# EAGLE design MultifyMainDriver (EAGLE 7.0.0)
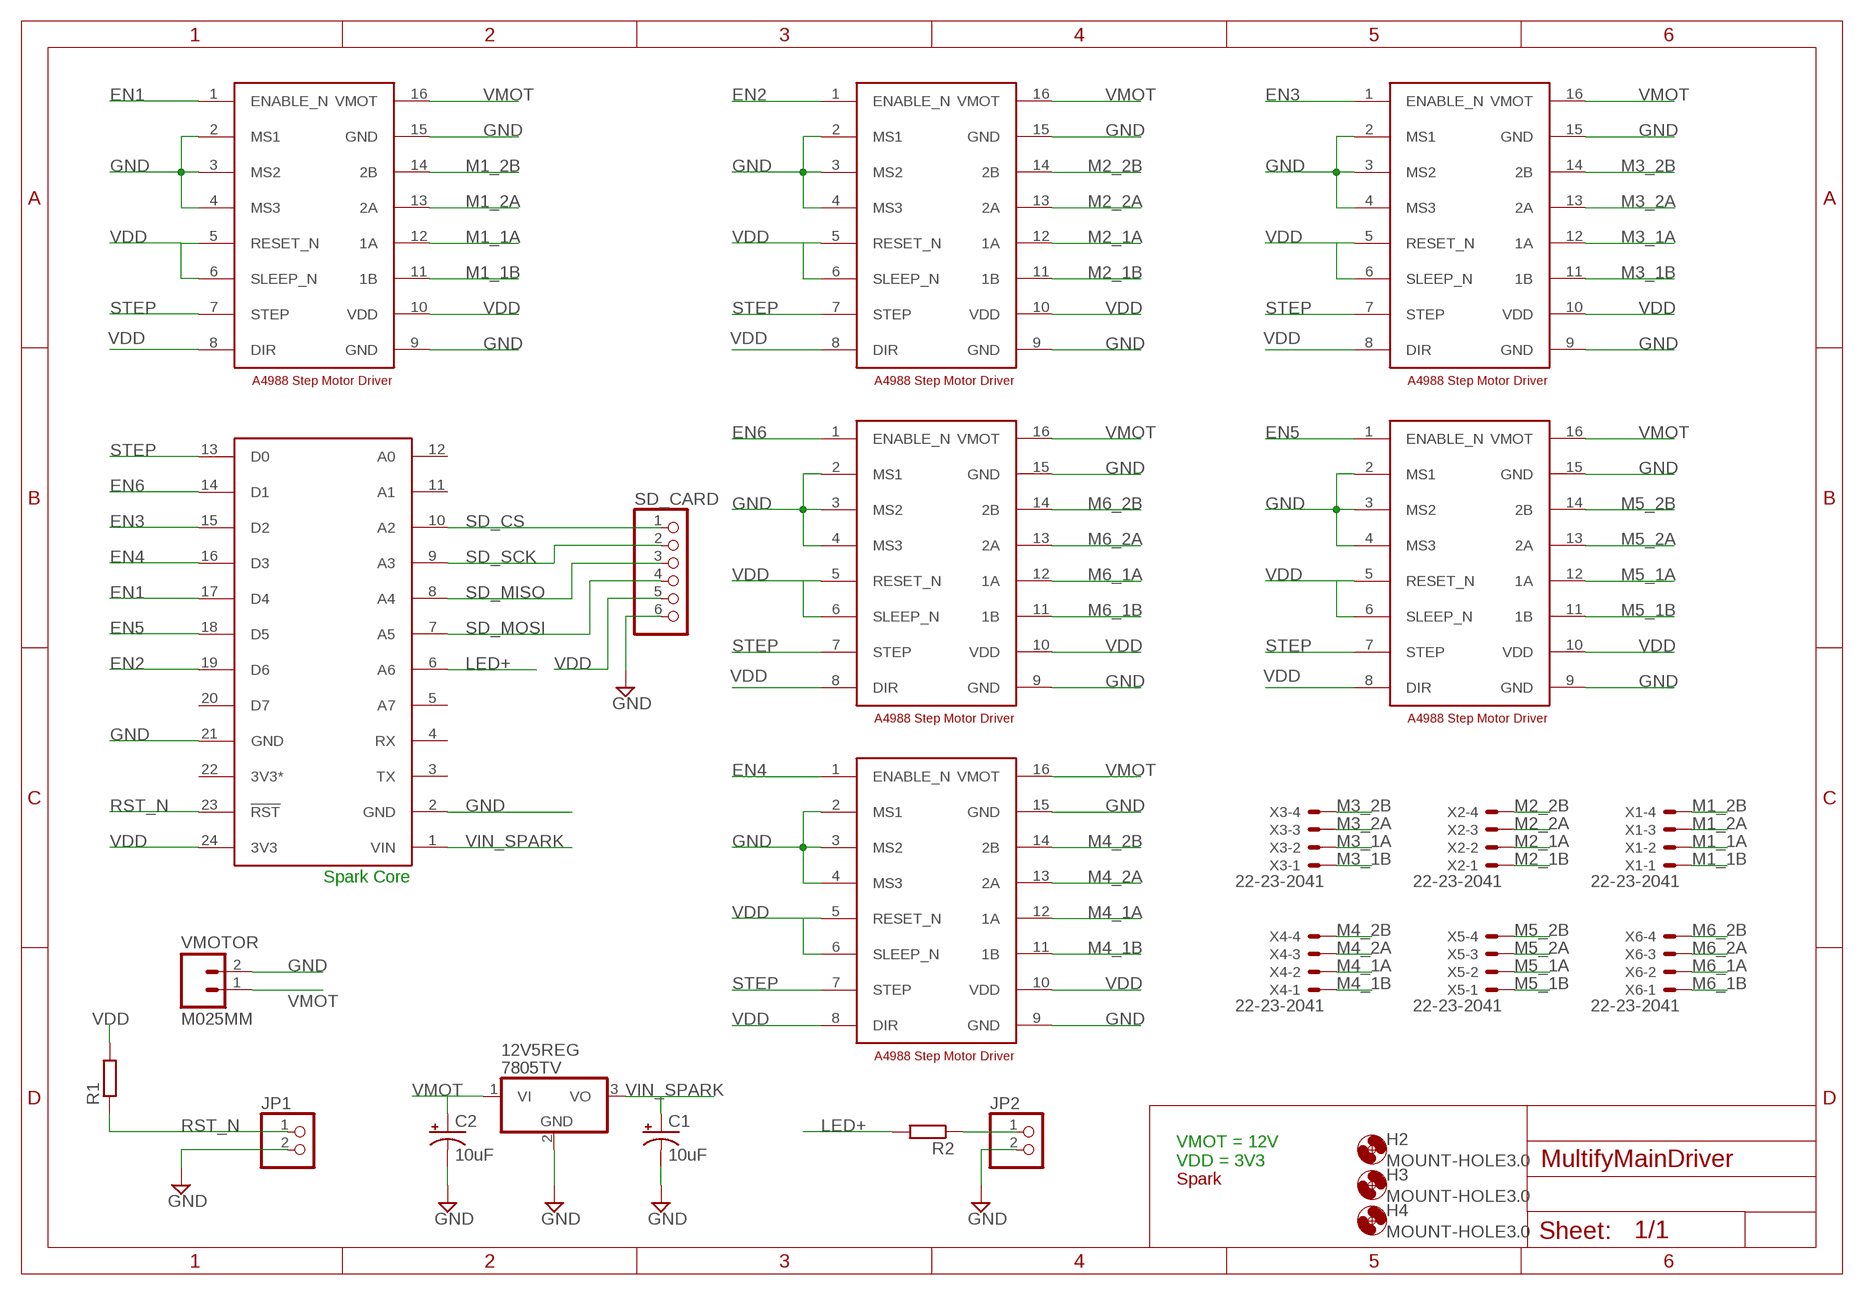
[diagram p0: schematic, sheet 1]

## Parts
12V5REG  7805TV  [TO220V]
C1  10uF  CPOL-USE3.5-8  [E3,5-8]
C2  10uF  CPOL-USE3.5-8  [E3,5-8]
DRIVER1  A4988_DEV  [A4988_PAC]
DRIVER2  A4988_DEV  [A4988_PAC]
DRIVER3  A4988_DEV  [A4988_PAC]
DRIVER4  A4988_DEV  [A4988_PAC]
DRIVER5  A4988_DEV  [A4988_PAC]
DRIVER6  A4988_DEV  [A4988_PAC]
H2  MOUNT-HOLE3.0  [3,0]
H3  MOUNT-HOLE3.0  [3,0]
H4  MOUNT-HOLE3.0  [3,0]
JP1  PINHD-1X2  [1X02]
JP2  PINHD-1X2  [1X02]
R1  R-EU_0207/7  [0207/7]
R2  R-EU_0207/7  [0207/7]
SD_CARD  PINHD-1X6  [1X06]
SPARK  SPARK_CORECORE  [SPARK_CORE]
U$2  SPARK_LOGO_WITH_PLANE  [SPARK_LOGO_PLUS_PLANE]
VMOTOR  M025MM  [SCREWTERMINAL-5MM-2]
X1  22-23-2041  [22-23-2041]
X2  22-23-2041  [22-23-2041]
X3  22-23-2041  [22-23-2041]
X4  22-23-2041  [22-23-2041]
X5  22-23-2041  [22-23-2041]
X6  22-23-2041  [22-23-2041]

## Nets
EN1: DRIVER1.1(ENABLE_N) SPARK.17(D4)
EN2: DRIVER2.1(ENABLE_N) SPARK.19(D6)
EN3: DRIVER3.1(ENABLE_N) SPARK.15(D2)
EN4: DRIVER4.1(ENABLE_N) SPARK.16(D3)
EN5: DRIVER6.1(ENABLE_N) SPARK.18(D5)
EN6: DRIVER5.1(ENABLE_N) SPARK.14(D1)
GND: 12V5REG.2(GND) C1.- C2.- DRIVER1.2(MS1) DRIVER1.3(MS2) DRIVER1.4(MS3) DRIVER1.9(GND) DRIVER1.15(GND) DRIVER2.2(MS1) DRIVER2.3(MS2) DRIVER2.4(MS3) DRIVER2.9(GND) DRIVER2.15(GND) DRIVER3.2(MS1) DRIVER3.3(MS2) DRIVER3.4(MS3) DRIVER3.9(GND) DRIVER3.15(GND) DRIVER4.2(MS1) DRIVER4.3(MS2) DRIVER4.4(MS3) DRIVER4.9(GND) DRIVER4.15(GND) DRIVER5.2(MS1) DRIVER5.3(MS2) DRIVER5.4(MS3) DRIVER5.9(GND) DRIVER5.15(GND) DRIVER6.2(MS1) DRIVER6.3(MS2) DRIVER6.4(MS3) DRIVER6.9(GND) DRIVER6.15(GND) JP1.2 JP2.2 SD_CARD.6 SPARK.2(GND) SPARK.21(GND) VMOTOR.2
LED+: R2.2 SPARK.6(A6)
M1_1A: DRIVER1.12(1A) X1.2
M1_1B: DRIVER1.11(1B) X1.1
M1_2A: DRIVER1.13(2A) X1.3
M1_2B: DRIVER1.14(2B) X1.4
M2_1A: DRIVER2.12(1A) X2.2
M2_1B: DRIVER2.11(1B) X2.1
M2_2A: DRIVER2.13(2A) X2.3
M2_2B: DRIVER2.14(2B) X2.4
M3_1A: DRIVER3.12(1A) X3.2
M3_1B: DRIVER3.11(1B) X3.1
M3_2A: DRIVER3.13(2A) X3.3
M3_2B: DRIVER3.14(2B) X3.4
M4_1A: DRIVER4.12(1A) X4.2
M4_1B: DRIVER4.11(1B) X4.1
M4_2A: DRIVER4.13(2A) X4.3
M4_2B: DRIVER4.14(2B) X4.4
M5_1A: DRIVER6.12(1A) X5.2
M5_1B: DRIVER6.11(1B) X5.1
M5_2A: DRIVER6.13(2A) X5.3
M5_2B: DRIVER6.14(2B) X5.4
M6_1A: DRIVER5.12(1A) X6.2
M6_1B: DRIVER5.11(1B) X6.1
M6_2A: DRIVER5.13(2A) X6.3
M6_2B: DRIVER5.14(2B) X6.4
N$1: JP2.1 R2.1
RST_N: JP1.1 R1.1 SPARK.23(!RST)
SD_CS: SD_CARD.1 SPARK.10(A2)
SD_MISO: SD_CARD.3 SPARK.8(A4)
SD_MOSI: SD_CARD.4 SPARK.7(A5)
SD_SCK: SD_CARD.2 SPARK.9(A3)
STEP: DRIVER1.7(STEP) DRIVER2.7(STEP) DRIVER3.7(STEP) DRIVER4.7(STEP) DRIVER5.7(STEP) DRIVER6.7(STEP) SPARK.13(D0)
VDD: DRIVER1.5(RESET_N) DRIVER1.6(SLEEP_N) DRIVER1.8(DIR) DRIVER1.10(VDD) DRIVER2.5(RESET_N) DRIVER2.6(SLEEP_N) DRIVER2.8(DIR) DRIVER2.10(VDD) DRIVER3.5(RESET_N) DRIVER3.6(SLEEP_N) DRIVER3.8(DIR) DRIVER3.10(VDD) DRIVER4.5(RESET_N) DRIVER4.6(SLEEP_N) DRIVER4.8(DIR) DRIVER4.10(VDD) DRIVER5.5(RESET_N) DRIVER5.6(SLEEP_N) DRIVER5.8(DIR) DRIVER5.10(VDD) DRIVER6.5(RESET_N) DRIVER6.6(SLEEP_N) DRIVER6.8(DIR) DRIVER6.10(VDD) R1.2 SD_CARD.5 SPARK.24(3V3)
VIN_SPARK: 12V5REG.3(VO) C1.+ SPARK.1(VIN)
VMOT: 12V5REG.1(VI) C2.+ DRIVER1.16(VMOT) DRIVER2.16(VMOT) DRIVER3.16(VMOT) DRIVER4.16(VMOT) DRIVER5.16(VMOT) DRIVER6.16(VMOT) VMOTOR.1
Unconnected: SPARK.3(TX) SPARK.4(RX) SPARK.5(A7) SPARK.11(A1) SPARK.12(A0) SPARK.20(D7)

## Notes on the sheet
- Spark Core
- VMOT = 12V
  VDD = 3V3

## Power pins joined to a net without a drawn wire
3V3*: SPARK.22(3V3*)

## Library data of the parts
12V5REG = linear:78*: Positive VOLTAGE REGULATOR Source: http://cache.national.com/ds/LM/LM78L05.pdf http://www.fairchildsemi.com/ds/LM/LM7805.pdf
C1 C2 = rcl:CPOL-US: POLARIZED CAPACITOR, American symbol
DRIVER1-DRIVER6 = A4988:A4988_DEV
H2-H4 = holes:MOUNT-HOLE: MOUNTING HOLE with drill center marker
JP1 JP2 = pinhead:PINHD-1X2: PIN HEADER
R1 R2 = rcl:R-EU_: RESISTOR, European symbol
SD_CARD = pinhead:PINHD-1X6: PIN HEADER
SPARK = Spark:SPARK_CORE
U$2 = Spark:SPARK_LOGO_WITH_PLANE
VMOTOR = SparkFun-Connectors:M02: Standard 2-pin 0.1" header. Use with; STOREFRONT_ID: PRT-08432
X1-X6 = con-molex:22-23-2041: .100" (2.54mm) Center Header - 4 Pin; MF: MOLEX; MPN: 22-23-2041; OC_FARNELL: 1462920; OC_NEWARK: 38C0355

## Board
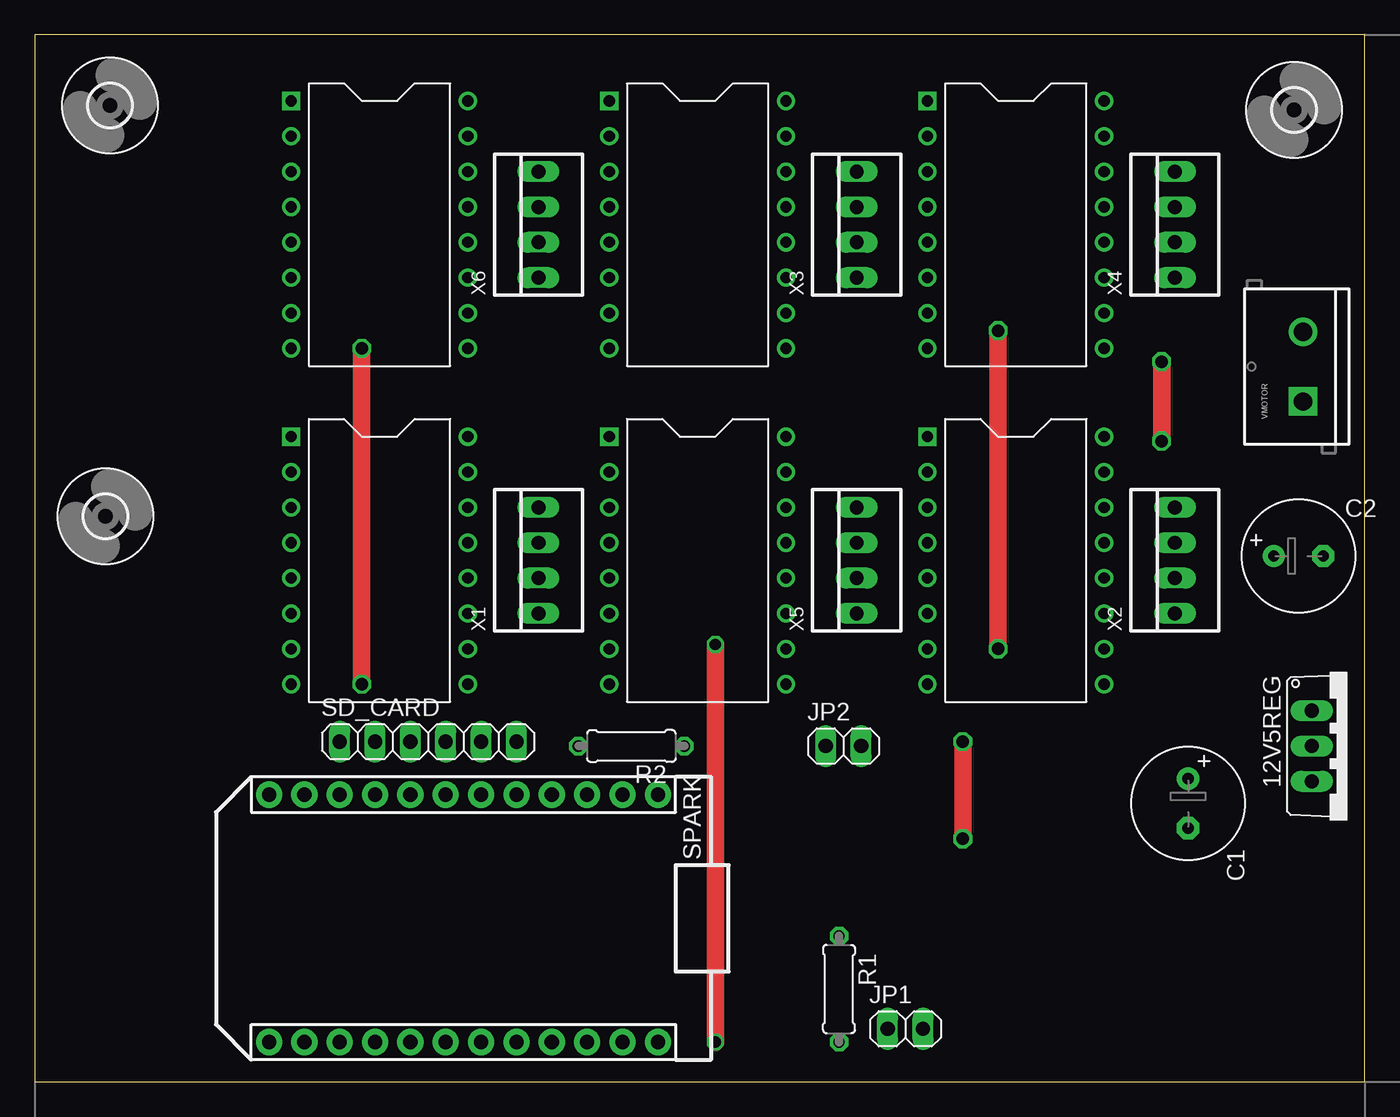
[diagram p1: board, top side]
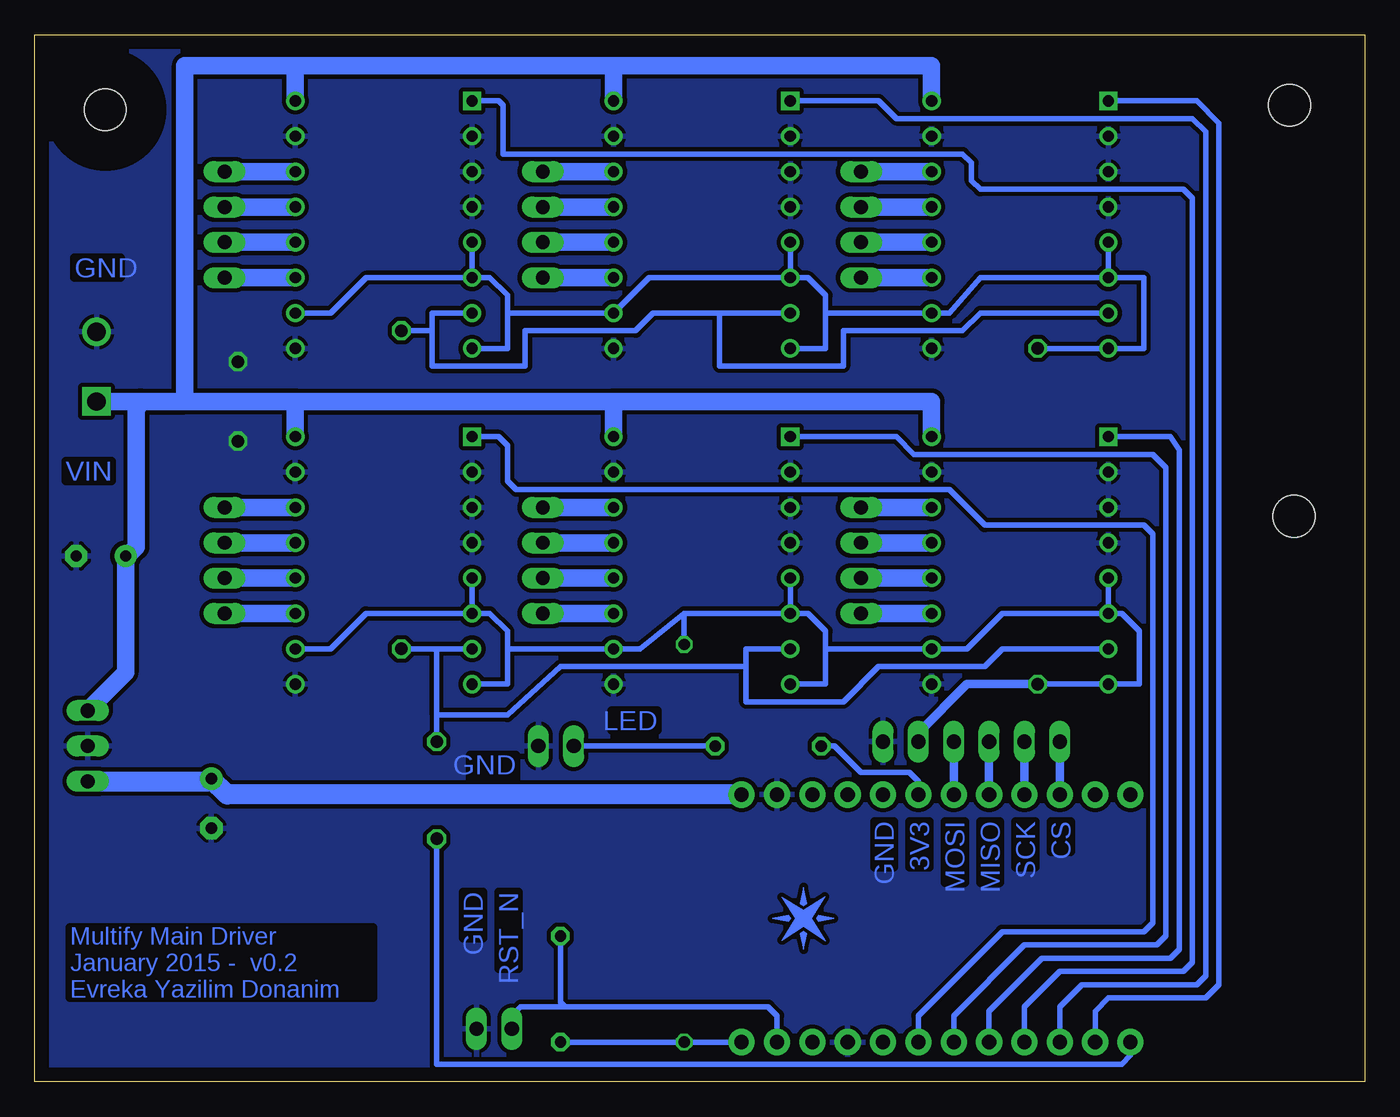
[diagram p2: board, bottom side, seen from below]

Size 95.56 x 75.24 mm. Coordinates in mm from the lower left corner, seen from the top.
Outline: 0,0 95.56,0 95.56,75.24 0,75.24 0,0
Copper layers (1*16): Top 0.035mm / dielectric 1.5mm / Bottom 0.035mm
Design rules "default": minimum track width 10mil, minimum drill 24mil, track to track 8mil, track to pad 8mil, pad to pad 8mil, via to via 8mil, smd to smd 8mil, copper to edge 40mil, drill to drill 8mil, minimum pad ring 10mil, minimum via ring 8mil, stop-mask expansion 4mil, vias tented up to drill 0mil, thermal gap 10mil

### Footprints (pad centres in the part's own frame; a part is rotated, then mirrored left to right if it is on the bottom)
TO220V = drill 1.016 long: 1 -2.54,-2.54; 2 0,-2.54; 3 2.54,-2.54
E3,5-8 = drill 0.813 pad 1.6: + -1.778,0 | drill 0.813 pad 1.6 octagon: - 1.778,0
A4988_PAC = drill 0.8 square: 1 -6.35,8.89 | drill 0.8: 2 -6.35,6.35; 3 -6.35,3.81; 4 -6.35,1.27; 5 -6.35,-1.27; 6 -6.35,-3.81; 7 -6.35,-6.35; 8 -6.35,-8.89; 9 6.35,-8.89; 10 6.35,-6.35; 11 6.35,-3.81; 12 6.35,-1.27; 13 6.35,1.27; 14 6.35,3.81; 15 6.35,6.35; 16 6.35,8.89
3,0 = hole 3: 0,0
1X02 = drill 1.016 long: 1 -1.27,0; 2 1.27,0
0207/7 = drill 0.813 octagon: 1 -3.81,0; 2 3.81,0
1X06 = drill 1.016 long: 1 -6.35,0; 2 -3.81,0; 3 -1.27,0; 4 1.27,0; 5 3.81,0; 6 6.35,0
SPARK_CORE = drill 1.016 pad 1.88: 1 -8.89,13.97; 2 -8.89,11.43; 3 -8.89,8.89; 4 -8.89,6.35; 5 -8.89,3.81; 6 -8.89,1.27; 7 -8.89,-1.27; 8 -8.89,-3.81; 9 -8.89,-6.35; 10 -8.89,-8.89; 11 -8.89,-11.43; 12 -8.89,-13.97; 13 8.89,-13.97; 14 8.89,-11.43; 15 8.89,-8.89; 16 8.89,-6.35; 17 8.89,-3.81; 18 8.89,-1.27; 19 8.89,1.27; 20 8.89,3.81; 21 8.89,6.35; 22 8.89,8.89; 23 8.89,11.43; 24 8.89,13.97
SCREWTERMINAL-5MM-2 = drill 1.3 pad 2.032 square: 1 0,0 | drill 1.3 pad 2.032: 2 5,0
22-23-2041 = drill 1 long: 1 -3.81,0; 2 -1.27,0; 3 1.27,0; 4 3.81,0

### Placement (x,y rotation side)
12V5REG  94.3,24.13 270 top
C1  82.87,20 270 top
C2  90.81,37.78 0 top
DRIVER1  24.77,37.47 0 top
DRIVER2  70.48,37.47 0 top
DRIVER3  47.62,61.59 0 top
DRIVER4  70.48,61.59 0 top
DRIVER5  24.77,61.59 0 top
DRIVER6  47.62,37.47 0 top
H2  90.49,69.85 0 top
H3  5.08,40.64 0 top
H4  5.4,70.17 0 top
JP1  62.55,3.81 0 top
JP2  58.1,24.13 0 top
R1  57.78,6.67 270 top
R2  42.86,24.13 180 top
SD_CARD  28.26,24.45 0 top
SPARK  30.8,11.75 270 top
U$2  40.32,11.75 0 bottom
VMOTOR  91.12,48.9 90 top
X1  36.2,37.47 90 top
X2  81.92,37.47 90 top
X3  59.05,61.59 90 top
X4  81.92,61.59 90 top
X5  59.05,37.47 90 top
X6  36.2,61.59 90 top

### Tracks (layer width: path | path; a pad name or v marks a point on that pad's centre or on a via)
EN1
  Bottom 0.406: DRIVER1.1 13.97,46.35 13.34,45.4 13.34,9.53 13.97,8.89 23.18,8.89 26.99,5.08 SPARK.17
EN2
  Bottom 0.406: SPARK.19 32.07,4.76 26.04,10.79 15.88,10.79 15.24,11.43 15.24,39.37 15.88,40.01 27.3,40.01 29.84,42.55 60.96,42.55 61.59,43.18 61.59,45.72 62.23,46.35 DRIVER2.1
EN3
  Bottom 0.406: DRIVER3.1 34.92,70.48 33.66,69.22 12.38,69.22 11.43,68.26 11.43,7.62 12.06,6.99 20.32,6.99 21.91,5.4 SPARK.15
EN4
  Bottom 0.406: DRIVER4.1 62.23,70.48 61.91,70.17 61.91,66.67 28.89,66.67 28.26,66.04 28.26,64.77 27.62,64.14 13.02,64.14 12.38,63.5 12.38,8.57 13.02,7.94 21.91,7.94 24.45,5.4 SPARK.16
EN5
  Bottom 0.406: DRIVER6.1 33.66,46.35 32.38,45.09 15.24,45.09 14.29,44.13 14.29,10.48 14.92,9.84 24.45,9.84 29.53,4.76 SPARK.18
EN6
  Bottom 0.406: 14.61,70.48 DRIVER5.1 12.06,70.48 10.48,68.9 10.48,6.99 11.43,6.03 18.41,6.03 19.37,5.08 SPARK.14
GND  (via drill 0.9)
  Top 1.27: v80.96,51.75 v80.96,46.04
  pour Bottom (isolate 0.305): 0.32,75.25 95.57,75.25 95.57,0 0.32,0
LED+
  Bottom 0.406: SPARK.6 32.07,21.59 32.7,22.23 36.2,22.23 38.1,24.13 R2.2
M1_1A
  Bottom 1.27: X1.2 DRIVER1.12
M1_1B
  Bottom 1.27: X1.1 DRIVER1.11
M1_2A
  Bottom 1.27: X1.3 DRIVER1.13
M1_2B
  Bottom 1.27: DRIVER1.14 X1.4
M2_1A
  Bottom 1.27: X2.2 DRIVER2.12
M2_1B
  Bottom 1.27: X2.1 DRIVER2.11
M2_2A
  Bottom 1.27: X2.3 DRIVER2.13
M2_2B
  Bottom 1.27: X2.4 DRIVER2.14
M3_1A
  Bottom 1.27: X3.2 DRIVER3.12
M3_1B
  Bottom 1.27: X3.1 DRIVER3.11
M3_2A
  Bottom 1.27: X3.3 DRIVER3.13
M3_2B
  Bottom 1.27: X3.4 DRIVER3.14
M4_1A
  Bottom 1.27: X4.2 DRIVER4.12
M4_1B
  Bottom 1.27: X4.1 DRIVER4.11
M4_2A
  Bottom 1.27: X4.3 DRIVER4.13
M4_2B
  Bottom 1.27: X4.4 DRIVER4.14
M5_1A
  Bottom 1.27: X5.2 DRIVER6.12
M5_1B
  Bottom 1.27: X5.1 DRIVER6.11
M5_2A
  Bottom 1.27: X5.3 DRIVER6.13
M5_2B
  Bottom 1.27: X5.4 DRIVER6.14
M6_1A
  Bottom 1.27: DRIVER5.12 X6.2
M6_1B
  Bottom 1.27: DRIVER5.11 X6.1
M6_2A
  Bottom 1.27: DRIVER5.13 X6.3
M6_2B
  Bottom 1.27: DRIVER5.14 X6.4
N$1
  Bottom 0.406: R2.1 JP2.1
RST_N
  Bottom 0.406: SPARK.23 42.23,4.76 42.86,5.4 57.47,5.4 | 57.47,5.4 60.64,5.4 61.28,4.76 JP1.1 | R1.1 57.78,5.71 57.47,5.4
SD_CS
  Bottom 0.61: SD_CARD.1 SPARK.10
SD_MISO
  Bottom 0.61: SD_CARD.3 SPARK.8
SD_MOSI
  Bottom 0.61: SD_CARD.4 SPARK.7
SD_SCK
  Bottom 0.61: SD_CARD.2 SPARK.9
STEP  (via drill 0.9)
  Top 1.27: v69.22,31.11 v69.22,53.98 | v66.67,24.45 v66.67,17.46
  Bottom 0.406: DRIVER6.7 44.45,31.11 44.45,29.84 | DRIVER5.7 27.62,55.24 28.89,53.98 37.47,53.98 37.47,51.44 46.35,51.44 46.35,55.24 | DRIVER3.7 46.35,55.24 | 46.35,55.24 51.12,55.24 52.39,53.98 60.33,53.98 60.33,51.44 66.99,51.44 66.99,53.98 | DRIVER4.7 66.99,55.24 66.99,53.98 | DRIVER1.7 26.04,31.11 27.3,29.84 34.92,29.84 37.47,27.3 44.45,27.3 44.45,29.84 | 44.45,29.84 57.78,29.84 61.59,26.35 66.67,26.35 | 66.67,26.35 66.67,31.11 | DRIVER2.7 66.67,31.11 | 66.67,31.11 v69.22,31.11 | v69.22,53.98 66.99,53.98 | SPARK.13 16.83,1.91 17.46,1.27 66.67,1.27 v66.67,17.46 | 66.67,26.35 v66.67,24.45
VDD  (via drill 0.8, 0.9)
  Top 1.27: v23.5,28.57 v23.5,52.7 | v48.9,2.86 v48.9,31.43
  Bottom 0.406: DRIVER5.5 DRIVER5.6 | DRIVER3.5 DRIVER3.6 | DRIVER4.5 DRIVER4.6 | DRIVER1.5 DRIVER1.6 | DRIVER6.5 DRIVER6.6 | DRIVER2.6 DRIVER2.5 | DRIVER2.10 74.3,31.11 71.75,33.66 DRIVER2.6 | DRIVER5.6 27.62,57.78 29.84,55.24 DRIVER5.10 38.73,55.24 | DRIVER3.6 51.44,57.78 DRIVER3.10 61.59,55.24 | DRIVER4.6 71.75,57.78 74.3,55.24 DRIVER4.10 | DRIVER6.6 48.9,33.66 | 48.9,33.66 52.07,31.11 DRIVER6.10 61.59,31.11 | DRIVER1.6 26.04,33.66 28.57,31.11 DRIVER1.10 38.73,31.11 | DRIVER5.6 15.88,57.78 15.88,52.7 DRIVER5.8 v23.5,52.7 | DRIVER3.8 38.73,52.7 38.73,55.24 | 38.73,55.24 38.73,56.52 40.01,57.78 DRIVER3.6 | DRIVER4.8 61.59,52.7 61.59,55.24 | 61.59,55.24 61.59,56.52 62.87,57.78 DRIVER4.6 | DRIVER1.6 17.46,33.66 16.19,32.38 16.19,28.57 DRIVER1.8 v23.5,28.57 | DRIVER6.8 38.73,28.57 38.73,31.11 | 38.73,31.11 38.73,32.38 40.01,33.66 DRIVER6.6 | DRIVER2.8 61.59,28.57 61.59,31.11 | 61.59,31.11 61.59,32.38 62.87,33.66 DRIVER2.6 | v48.9,31.43 48.9,33.66 | SPARK.24 v48.9,2.86 R1.2
  Bottom 0.61: SD_CARD.5 32.07,25.08 28.57,28.57 v23.5,28.57
VIN_SPARK
  Bottom 1.422: SPARK.1 81.72,20.64 C1.+ 83.06,21.59 12V5REG.3
VMOT
  Bottom 1.27: DRIVER5.16 31.11,73.03 53.98,73.03 | 53.98,73.03 DRIVER3.16 | DRIVER4.16 76.83,73.03 | 76.83,73.03 53.98,73.03 | DRIVER1.16 31.11,48.9 53.98,48.9 | 53.98,48.9 DRIVER6.16 | DRIVER2.16 76.83,48.9 | 76.83,48.9 53.98,48.9 | 76.83,48.9 84.77,48.9 | 84.77,48.9 84.77,73.03 76.83,73.03 | VMOTOR.1 87.95,48.9 | 87.95,48.9 84.77,48.9 | 87.95,48.9 88.27,48.26 88.27,38.42 88.9,37.78 C2.+ 89.03,29.4 12V5REG.1

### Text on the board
Bottom: GND | VIN | LED | GND | CS | SCK | MISO | MOSI | 3V3 | GND | RST_N | GND | Multify Main Driver / January 2015 - v0.2 / Evreka Yazilim Donanim

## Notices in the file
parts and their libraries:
SparkFun-Connectors: Licensing: Creative Commons ShareAlike 4.0 International - https://creativecommons.org/licenses/by-sa/4.0
